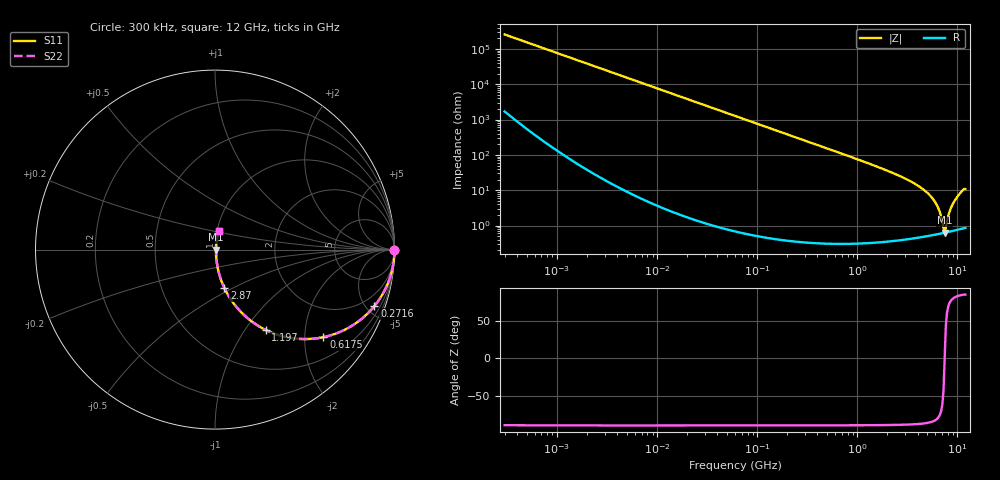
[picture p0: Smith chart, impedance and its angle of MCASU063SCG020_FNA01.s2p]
! MCASU063SCG020_FNA01  S-PARAMETER MODEL  ( Standard Model )
! Model Generated by TAIYO YUDEN Corporation (http://www.ty-top.com)
! Version 1.0
! TAIYO YUDEN Control No. 230609
! Copyright(c) 2023 TAIYO YUDEN CO.,LTD. All Rights Reserved.
! Product Description (link to TY-COMPAS)
! https://ds.yuden.co.jp/TYCOMPAS/or/detail?pn=MCASU063SCG020BFNA01&u=M
! Products Name : Multilayer Ceramic Capacitors
! Characteristics :
!  Capacitance : 2 [pF] , Rated Voltage : 50 [V] , TCC : CG / C0G
!  Case Size : 0.6 x 0.3 / 0.024 x 0.012 [mm/inch] , Thickness : 0.3 / 0.012 [mm/inch]
!  (Conditions: Temperature = 25 [degC] , DC Bias Voltage = 0 [V])
! External Node Assignments :
!  1  o---| |---o  2
! GND o---------o GND
! Frequency Range : 0.3MHz  -  12000MHz  [ 401 STEP ]
# MHZ S RI R 50
! Freq[MHz].  S11 Real  S11 Imag  S21 Real  S21 Imag  S12 Real  S12 Imag  S22 Real  S22 Imag
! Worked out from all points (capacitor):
!   401 points, 300 kHz to 12 GHz, reference 50 ohm
!   read as one part in series: C = 2.07 pF near 316.3 kHz
!   lowest |Z| = 628 mohm at 7.449 GHz (marker M1)
!   series resonance near 7.448 GHz, so ESL is about 220 pH
!   S11 on the Smith chart (normalised r, x): 300 kHz: open; 271.6 MHz: 1.01, -5.64; 617.5 MHz: 1.01, -2.47; 1.197 GHz: 1.01, -1.25; 2.87 GHz: 1.01, -0.46; 12 GHz: 1.02, +0.22
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0.3  1 -0.000391  2.74e-06 0.000391  2.74e-06 0.000391  1 -0.000391
1.769972  1 -0.00231  7.79e-06 0.00231  7.79e-06 0.00231  1 -0.00231
10.44266  0.9998 -0.0136  0.000192 0.0136  0.000192 0.0136  0.9998 -0.0136
60  0.9939 -0.0777  0.00612 0.0777  0.00612 0.0777  0.9939 -0.0777
132.8329  0.9708 -0.1681  0.0292 0.1681  0.0292 0.1681  0.9708 -0.1681
271.6094  0.8881 -0.3146  0.1119 0.3146  0.1119 0.3146  0.8881 -0.3146
353.9943  0.8235 -0.3805  0.1765 0.3805  0.1765 0.3805  0.8235 -0.3805
617.4538  0.6035 -0.4879  0.3965 0.4879  0.3965 0.4879  0.6035 -0.4879
1197.383  0.2815 -0.4472  0.7185 0.4472  0.7185 0.4472  0.2815 -0.4472
2088.533  0.1054 -0.3019  0.8946 0.3019  0.8946 0.3019  0.1054 -0.3019
2870.14  0.0527 -0.215  0.9473 0.215  0.9473 0.215  0.0527 -0.215
4158.869  0.0203 -0.1241  0.9797 0.1241  0.9797 0.1241  0.0203 -0.1241
5420.343  0.00961 -0.0659  0.9904 0.0659  0.9904 0.0659  0.00961 -0.0659
6354.153  0.00677 -0.0328  0.9932 0.0328  0.9932 0.0328  0.00677 -0.0328
6699.894  0.00635 -0.022  0.9937 0.022  0.9937 0.022  0.00635 -0.022
7064.448  0.00617 -0.0112  0.9938 0.0112  0.9938 0.0112  0.00617 -0.0112
7448.838  0.00624 1.19e-05  0.9938 -1.19e-05  0.9938 -1.19e-05  0.00624 1.19e-05
7648.807  0.00638 0.00587  0.9936 -0.00587  0.9936 -0.00587  0.00638 0.00587
8503.825  0.00755 0.0277  0.9925 -0.0277  0.9925 -0.0277  0.00755 0.0277
9207.246  0.00919 0.0452  0.9908 -0.0452  0.9908 -0.0452  0.00919 0.0452
10793.46  0.0152 0.0844  0.9848 -0.0844  0.9848 -0.0844  0.0152 0.0844
12000  0.0198 0.105  0.9802 -0.105  0.9802 -0.105  0.0198 0.105
